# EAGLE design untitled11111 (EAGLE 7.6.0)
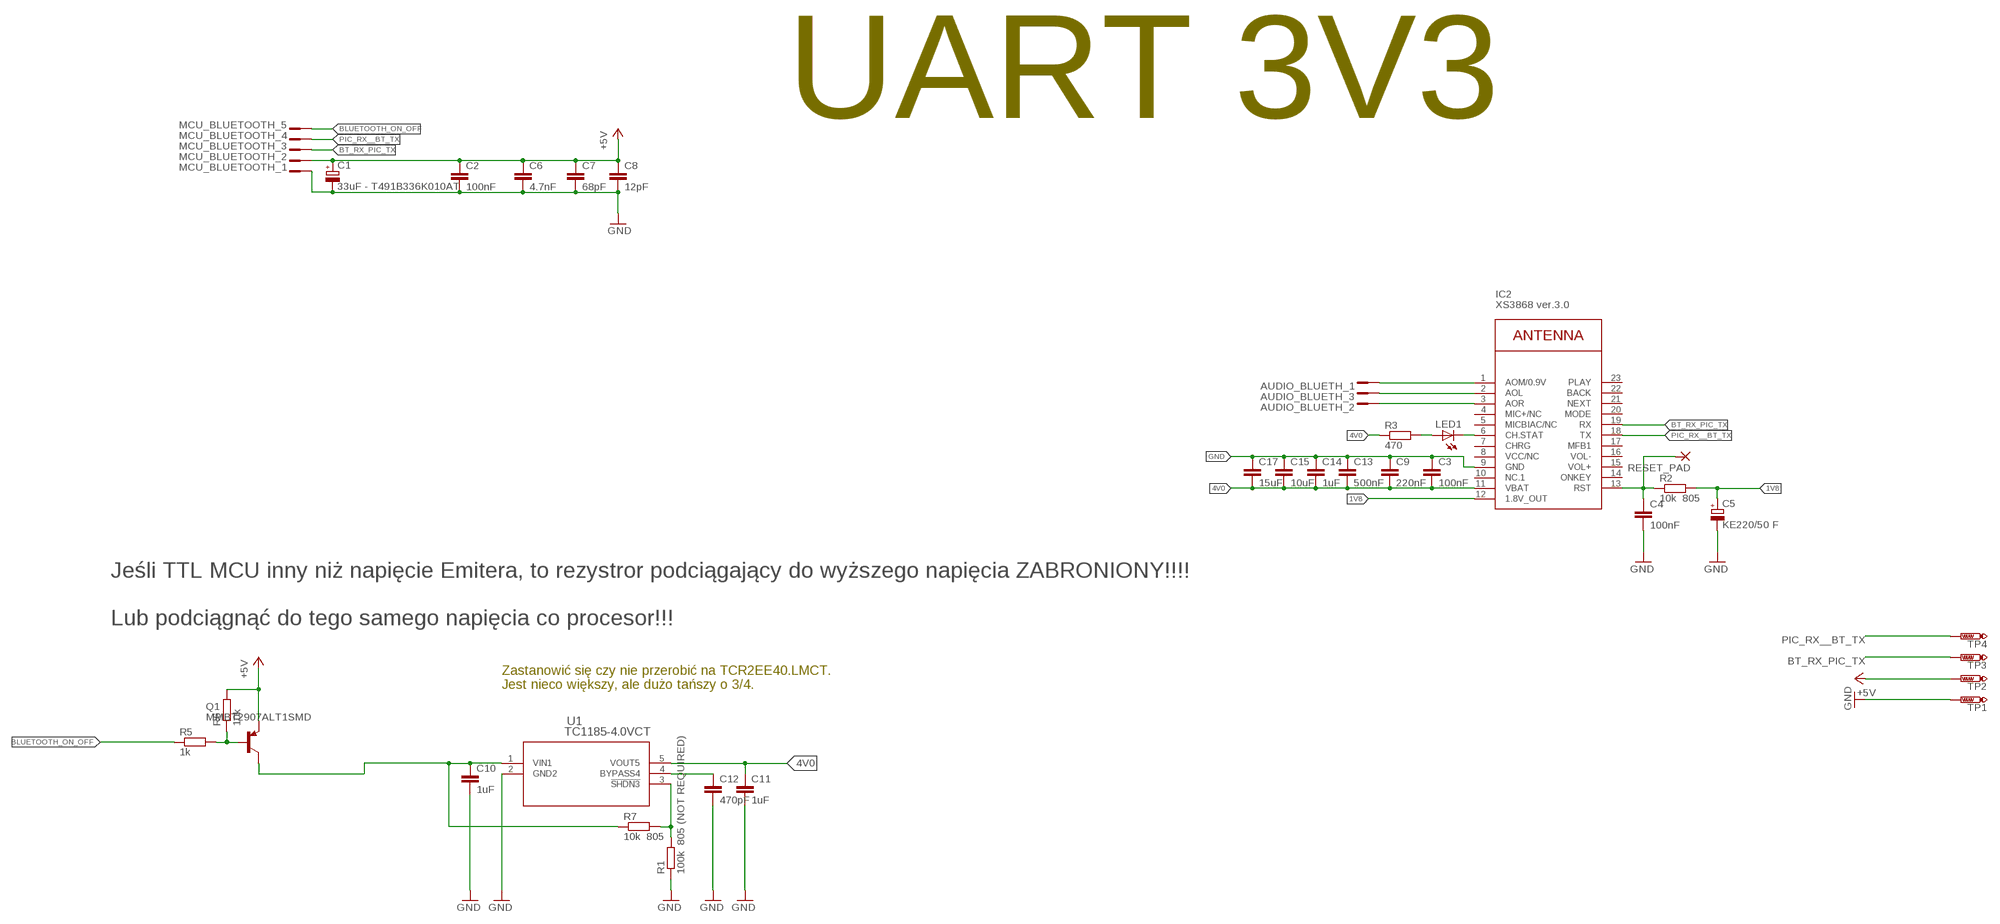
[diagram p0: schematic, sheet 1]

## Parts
AUDIO_BLUETH  JST_3_PIN_B3B-PH-KS  [B3B-PH-KS]
C1  33uF - T491B336K010AT  CPOL-EUSMCC  [SMC_C]
C2  100nF  C-EUC0805  [C0805]
C3  100nF  C-EUC0805  [C0805]
C4  100nF  C-EUC0805  [C0805]
C5  KE220/50 F  CPOL-EUG  [PANASONIC_G]
C6  4.7nF  C-EUC0805  [C0805]
C7  68pF  C-EUC0805  [C0805]
C8  12pF  C-EUC0805  [C0805]
C9  220nF  C-EUC0805  [C0805]
C10  1uF  C-EUC0805  [C0805]
C11  1uF  C-EUC0805  [C0805]
C12  470pF  C-EUC0805  [C0805]
C13  500nF  C-EUC0805  [C0805]
C14  1uF  C-EUC0805  [C0805]
C15  10uF  C-EUC0805  [C0805]
C17  15uF  C-EUC0805  [C0805]
IC2  XS3868 ver.3.0  WIRELESS-BLUETOOTH-XS3868  [WIRELESS-BLUETOOTH-XS3868]
LED1  LEDSML0805  [SML0805]
MCU_BLUETOOTH  JST_5_PIN_B5B-PH-KS  [B5B-PH-KS]
Q1  MMBT2907ALT1SMD  [SOT23-BEC]
R1  100k 805 (NOT REQUIRED)  R-EU_M0805  [M0805]
R2  10k 805  R-EU_M0805  [M0805]
R3  470  R-EU_M0805  [M0805]
R5  1k  R-EU_M0805  [M0805]
R6  10k  R-EU_M0805  [M0805]
R7  10k 805  R-EU_M0805  [M0805]
RESET_PAD  SMD2  [SMD1,27-2,54]
TP1  PTR1B1,27  [B1,27]
TP2  PTR1B1,27  [B1,27]
TP3  PTR1B1,27  [B1,27]
TP4  PTR1B1,27  [B1,27]
U1  TC1185-4.0VCT  TC1185-X.XXCT713SOT-23-5_MC-M  [SOT-23-5_MC-M]

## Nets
1V8: C5.+ IC2.12(1.8V_OUT) R2.2
4V0: C3.2 C9.2 C11.1 C13.2 C14.2 C15.2 C17.2 IC2.11(VBAT) R3.1 U1.5(VOUT5)
5V0_BLUETOOTH_ENABLED: C10.1 Q1.C R7.1 U1.1(VIN1)
+5V: C1.+ C2.1 C6.1 C7.1 C8.1 MCU_BLUETOOTH.P$2 Q1.E R6.2 TP2.TP
AUDIO_DIFF_COMMON: AUDIO_BLUETH.P$1 IC2.1(AOM/0.9V)
BLUETOOTH_ON_OFF: MCU_BLUETOOTH.P$5 R5.1
BT_LED: IC2.6(CH.STAT) LED1.C
BT_RX_PIC_TX: IC2.19(RX) MCU_BLUETOOTH.P$3 TP3.TP
BTOUT_LEFT: AUDIO_BLUETH.P$2 IC2.3(AOR)
BTOUT_RIGHT: AUDIO_BLUETH.P$3 IC2.2(AOL)
GND: C1.- C2.2 C3.1 C4.2 C5.- C6.2 C7.2 C8.2 C9.1 C10.2 C11.2 C12.2 C13.1 C14.1 C15.1 C17.1 IC2.9(GND) MCU_BLUETOOTH.P$1 R1.1 TP1.TP U1.2(GND2)
N$2: Q1.B R5.2 R6.1
N$4: C12.1 U1.4(BYPASS4)
N$5: LED1.A R3.2
N$6: R1.2 R7.2 U1.3(!SHDN3)
PIC_RX__BT_TX: IC2.18(TX) MCU_BLUETOOTH.P$4 TP4.TP
RST: C4.1 IC2.13(RST) R2.1 RESET_PAD.1(P)
Unconnected: IC2.4(MIC+/NC) IC2.5(MICBIAC/NC) IC2.7(CHRG) IC2.8(VCC/NC) IC2.10(NC.1) IC2.14(ONKEY) IC2.15(VOL+) IC2.16(VOL-) IC2.17(MFB1) IC2.20(MODE) IC2.21(NEXT) IC2.22(BACK) IC2.23(PLAY)

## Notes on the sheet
- UART 3V3
- Jeśli TTL MCU inny niż napięcie Emitera, to rezystror podciągający do wyższego napięcia ZABRONIONY!!!!
  
  Lub podciągnąć do tego samego napięcia co procesor!!!
- Zastanowić się czy nie przerobić na TCR2EE40.LMCT.
  Jest nieco większy, ale dużo tańszy o 3/4.

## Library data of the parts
AUDIO_BLUETH = conn-JST:JST_3_PIN_
C1 = resistor:CPOL-EU: POLARIZED CAPACITOR, European symbol
C2-C4 C6-C15 C17 = resistor:C-EU: CAPACITOR, European symbol
C5 = rcl:CPOL-EU: POLARIZED CAPACITOR, European symbol
IC2 = diy-modules:WIRELESS-BLUETOOTH-XS3868: Bluetooth Stereo Audio Module based on OVC3860 chip More details available here: http://artofcircuits.com/product/bluetooth-2-0-edr-stereo-audio-ovc3860-module-model-xs-3868 Click here to find device on ebay.com
LED1 = led:LED: LED
MCU_BLUETOOTH = conn-JST:JST_5_PIN_
Q1 = transistor-pnp:MMBT2907*: PNP Transistror
R1-R3 R5-R7 = rcl:R-EU_: RESISTOR, European symbol
RESET_PAD = wirepad:SMD2: SMD PAD
TP1-TP4 = testpad:PTR1: TEST PIN
U1 = TC1185:TC1185-X.XXCT713; MANUFACTURER_PART_NUMBER: TC1185X.XXCT713; VENDOR: Microchip

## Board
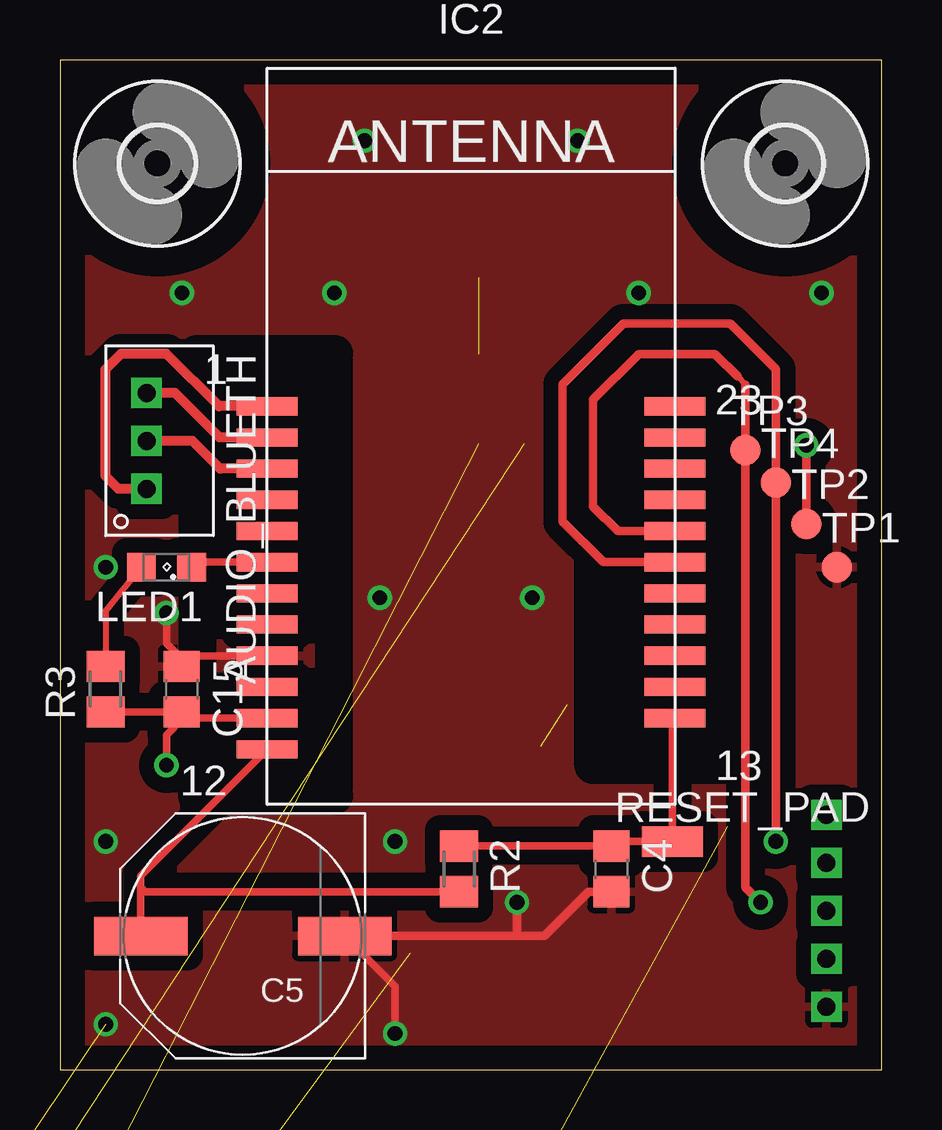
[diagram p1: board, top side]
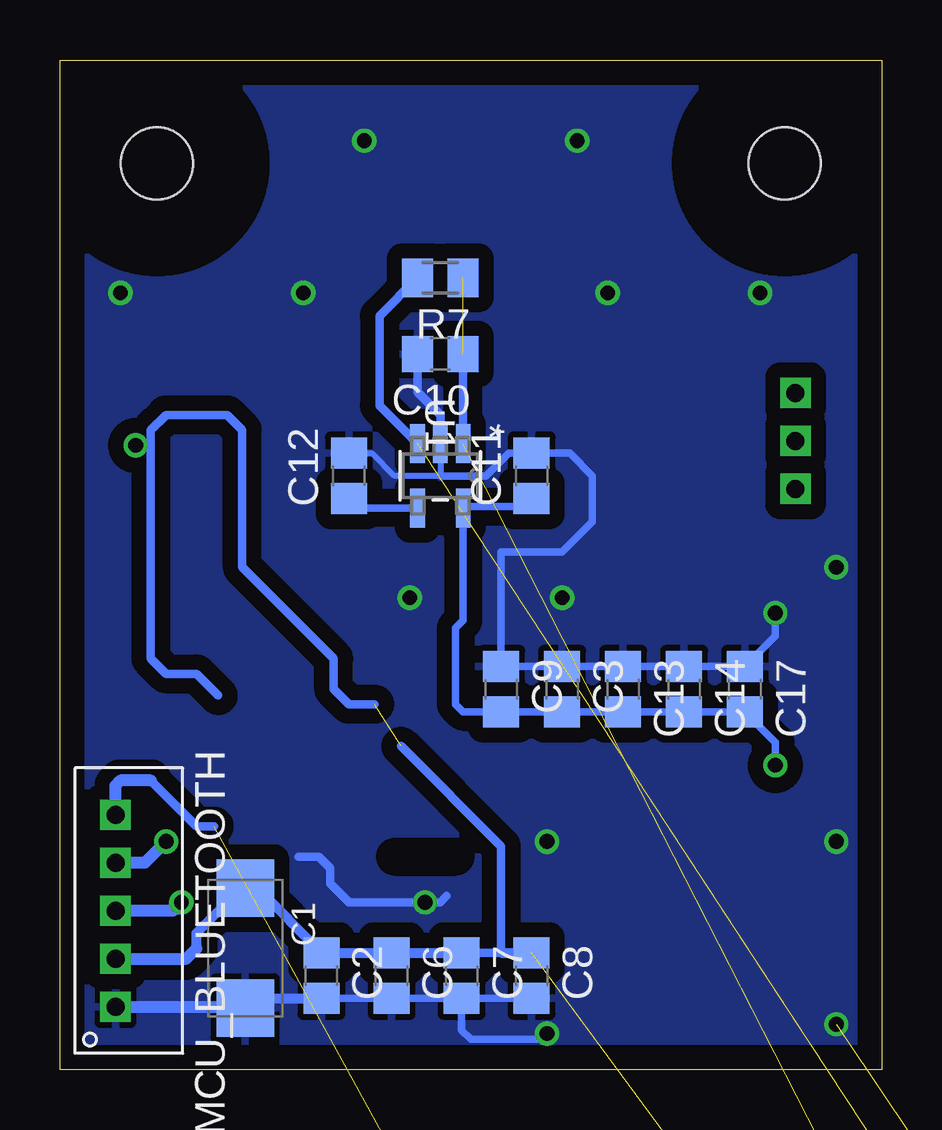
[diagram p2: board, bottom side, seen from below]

Size 34.27 x 42.1 mm. Coordinates in mm from the lower left corner, seen from the top.
Outline: 0,0 34.27,0 34.27,42.1 0,42.1 0,0
Copper layers (1*16): Top 0.035mm / dielectric 1.5mm / Bottom 0.035mm
Design rules "default": minimum track width 10mil, minimum drill 24mil, track to track 8mil, track to pad 8mil, pad to pad 8mil, via to via 8mil, smd to smd 8mil, copper to edge 40mil, drill to drill 8mil, minimum pad ring 10mil, minimum via ring 8mil, stop-mask expansion 4mil, vias tented up to drill 0mil, thermal gap 10mil
tRestrict: 8 lines
bRestrict: area 17.8,8.9 to 20.3,8.9

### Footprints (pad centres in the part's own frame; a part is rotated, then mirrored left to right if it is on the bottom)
B3B-PH-KS = drill 0.75 pad 1.2 square: P$1 -2,1.7; P$2 -4,1.7; P$3 -6,1.7
SMC_C = smd 2.4 x 2.4: + -2.5,0; - 2.5,0
C0805 = smd 1.3 x 1.5: 1 -0.95,0; 2 0.95,0
PANASONIC_G = smd 3.9 x 1.6: + 4.25,0; - -4.25,0
WIRELESS-BLUETOOTH-XS3868 = smd 2.54 x 0.762: 1 -8.5,0.995; 2 -8.5,-0.305; 3 -8.5,-1.605; 4 -8.5,-2.905; 5 -8.5,-4.205; 6 -8.5,-5.505; 7 -8.5,-6.805; 8 -8.5,-8.105; 9 -8.5,-9.405; 10 -8.5,-10.705; 11 -8.5,-12.005; 12 -8.5,-13.305; 13 8.5,-12.005; 14 8.5,-10.705; 15 8.5,-9.405; 16 8.5,-8.105; 17 8.5,-6.805; 18 8.5,-5.505; 19 8.5,-4.205; 20 8.5,-2.905; 21 8.5,-1.605; 22 8.5,-0.305; 23 8.5,0.995
SML0805 = smd 1.2 x 1.2: A 1.05,0; C -1.05,0
B5B-PH-KS = drill 0.75 pad 1.2 square: P$1 -2,1.7; P$2 -4,1.7; P$3 -6,1.7; P$4 -8,1.7; P$5 -10,1.7
SOT23-BEC = smd 1 x 1.4: B -0.95,-1.1; C 0,1.1; E 0.95,-1.1
M0805 = smd 1.3 x 1.6: 1 -0.95,0; 2 0.95,0
SMD1,27-2,54 = smd 1.27 x 2.54: 1 0,0
B1,27 = smd 1.27 x 1.27: TP 0,0
SOT-23-5_MC-M = smd 1.626 x 0.61: 1 -1.346,0.95; 2 -1.346,0; 3 -1.346,-0.95; 4 1.346,-0.95; 5 1.346,0.95
3,0 = hole 3: 0,0

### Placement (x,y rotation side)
AUDIO_BLUETH  1.9,22.23 270 top
C1  26.54,5.08 270 bottom
C2  23.37,3.94 270 bottom
C3  13.33,15.88 270 bottom
C4  22.99,8.38 270 top
C5  7.62,5.59 180 top
C6  20.45,3.94 270 bottom
C7  17.53,3.94 270 bottom
C8  14.6,3.94 270 bottom
C9  15.87,15.88 270 bottom
C10  18.41,29.84 180 bottom
C11  14.6,24.77 90 bottom
C12  22.23,24.77 90 bottom
C13  10.79,15.88 270 bottom
C14  8.26,15.88 270 bottom
C15  5.08,15.88 270 top
C17  5.71,15.88 270 bottom
IC2  17.14,26.67 0 top
LED1  4.44,20.96 180 top
MCU_BLUETOOTH  33.65,0.63 270 bottom
Q1  not placed on the board
R1  not placed on the board
R2  16.64,8.38 270 top
R3  1.9,15.88 90 top
R5  not placed on the board
R6  not placed on the board
R7  18.41,33.02 180 bottom
RESET_PAD  25.53,9.52 270 top
TP1  32.38,20.96 0 top
TP2  31.11,22.77 0 top
TP3  28.57,25.85 0 top
TP4  29.84,24.48 0 top
U1  18.41,24.77 270 bottom
U$2  [3,0]  4.06,37.78 0 top
U$3  [3,0]  30.23,37.78 0 top

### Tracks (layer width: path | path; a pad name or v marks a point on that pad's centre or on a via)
1V8
  Top 0.305: IC2.12 3.37,8.09 3.37,7.62 | 3.37,7.62 C5.+ | R2.2 3.56,7.43 3.37,7.62
4V0  (via drill 0.61)
  Top 0.305: C15.2 R3.1 | IC2.11 5.34,14.66 C15.2 | C15.2 5.08,14.61 4.44,13.97 v4.44,12.7
  Bottom 0.305: C17.2 5.4,14.93 | C17.2 C14.2 C13.2 C3.2 C9.2 17.46,14.93 17.78,15.24 17.78,18.41 17.46,18.73 U1.5 17.39,23.5 14.6,23.5 C11.1 | v4.44,12.7 4.44,13.66 C17.2
5V0_BLUETOOTH_ENABLED  (2 unrouted)
  Bottom 0.356: U1.1 C10.1
+5V  (via drill 0.61)  (3 unrouted)
  Top 0.356: TP2.TP v31.11,26.04
  Bottom 0.356: 21.16,15.24 22.23,15.24 22.86,15.88 22.86,17.14 26.67,20.96 26.67,26.67 27.3,27.3 29.84,27.3 30.48,26.67 30.48,26.04 | 20.05,13.51 15.87,9.32 15.87,4.89 C7.1 | 15.02,5.3 C8.1 | 30.48,26.04 30.48,17.14 29.84,16.51 28.57,16.51 27.67,15.61 | v31.11,26.04 30.48,26.04
  Bottom 0.406: C7.1 C6.1 C2.1 | C2.1 23.85,4.89 | C2.1 26.06,7.58 C1.+ 26.54,7.09 27.2,7.09 28.57,5.72 28.57,5.06 | 15.87,4.89 C8.1
  Bottom 0.508: MCU_BLUETOOTH.P$2 29,4.63 28.57,5.06
AUDIO_DIFF_COMMON
  Top 0.406: IC2.1 6.62,27.66 4.44,29.84 2.54,29.84 1.9,29.21 1.9,24.77 2.44,24.23 AUDIO_BLUETH.P$1
BLUETOOTH_ON_OFF  (1 unrouted)
  Bottom 0.356: 27.84,10.16 28.57,10.16 30.48,12.07
  Bottom 0.508: 30.48,12.07 31.75,12.07 31.95,11.86 MCU_BLUETOOTH.P$5
BT_LED
  Top 0.305: LED1.C 5.71,21.16 IC2.6
BT_RX_PIC_TX  (via drill 0.61)
  Top 0.254: TP3.TP 28.57,28.57 28.26,28.89
  Top 0.356: IC2.19 23.26,22.46 22.23,23.5 22.23,27.94 24.13,29.84 27.3,29.84 28.26,28.89 | 28.57,28.57 28.57,7.62 v29.21,6.99
  Bottom 0.508: v29.21,6.99 29.56,6.64 MCU_BLUETOOTH.P$3
BTOUT_LEFT
  Top 0.406: IC2.3 6.68,25.07 5.52,26.23 AUDIO_BLUETH.P$2
BTOUT_RIGHT
  Top 0.406: IC2.2 6.65,26.37 4.79,28.23 AUDIO_BLUETH.P$3
GND  (via drill 0.61)  (1 unrouted)
  Top 0.305: IC2.9 5.52,17.27 C15.1 5.08,17.14 4.44,17.78 v4.44,19.05 | 12.06,5.39 C5.- 13.97,3.49 v13.97,1.52
  Top 0.356: C4.2 22.04,7.43 20.19,5.59 19.05,5.59 | 19.05,5.59 C5.- | v19.05,6.99 19.05,5.59
  Bottom 0.254: U1.2 18.41,24.77 20.32,24.77 21.27,25.71 C12.2
  Bottom 0.305: C2.2 C6.2 C7.2 | C17.1 C14.1 C13.1 C3.1 C9.1 15.87,21.59 13.33,21.59 12.06,22.86 12.06,24.77 13.01,25.71 C11.2 15.56,25.71 16.51,24.77 18.41,24.77 | C17.1 5.39,17.14 | v4.44,19.05 4.44,18.1 C17.1 | C7.2 C8.2 | C7.2 17.53,1.65 17.14,1.27 14.22,1.27 v13.97,1.52
  Bottom 0.356: U1.2 18.41,27.3 19.37,28.26 C10.2 | 18.15,7.25 18.41,6.99 v19.05,6.99 22.23,6.99 23.01,7.77 23.01,8.43 23.48,8.89 24.33,8.89
  Bottom 0.406: C2.2 25.53,2.99 C1.- 26.79,2.63
  Bottom 0.508: MCU_BLUETOOTH.P$1 26.79,2.63
  other vias: 5.08,32.38 31.75,32.38 1.9,1.91 1.9,9.52 13.97,9.52 11.43,32.38 24.13,32.38 13.33,19.69 19.69,19.69 12.7,38.73 21.59,38.73 1.9,20.96
  pour Bottom (isolate 0.635): -1.91,24.13 -1.91,43.18 36.2,43.18 36.2,-1.27 -0.64,-1.27 -1.91,-1.27
  pour Top (isolate 0.635): -1.91,22.86 -1.91,43.18 36.2,43.18 36.2,-1.27 -1.91,-1.27
N$2  (2 unrouted)
N$4
  Bottom 0.305: U1.4 21.83,23.42 C12.1
N$5
  Top 0.254: LED1.A 1.9,19.14 R3.2
N$6  (1 unrouted)
  Bottom 0.356: R7.2 20.95,31.43 20.95,27.7 U1.3
PIC_RX__BT_TX  (via drill 0.61)
  Top 0.254: TP4.TP 29.84,29.21
  Top 0.356: IC2.18 22.65,21.16 20.95,22.86 20.95,28.57 23.49,31.12 27.94,31.12 29.84,29.21 v29.84,9.52
  Bottom 0.508: v29.84,9.52 30.73,8.64 MCU_BLUETOOTH.P$4
RST
  Top 0.305: IC2.13 25.53,14.66 RESET_PAD.1 23.18,9.52 C4.1 R2.1

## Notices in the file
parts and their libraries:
diy-modules: Released under the Creative Commons Attribution 4.0 International License: http://creativecommons.org/licenses/by/4.0
